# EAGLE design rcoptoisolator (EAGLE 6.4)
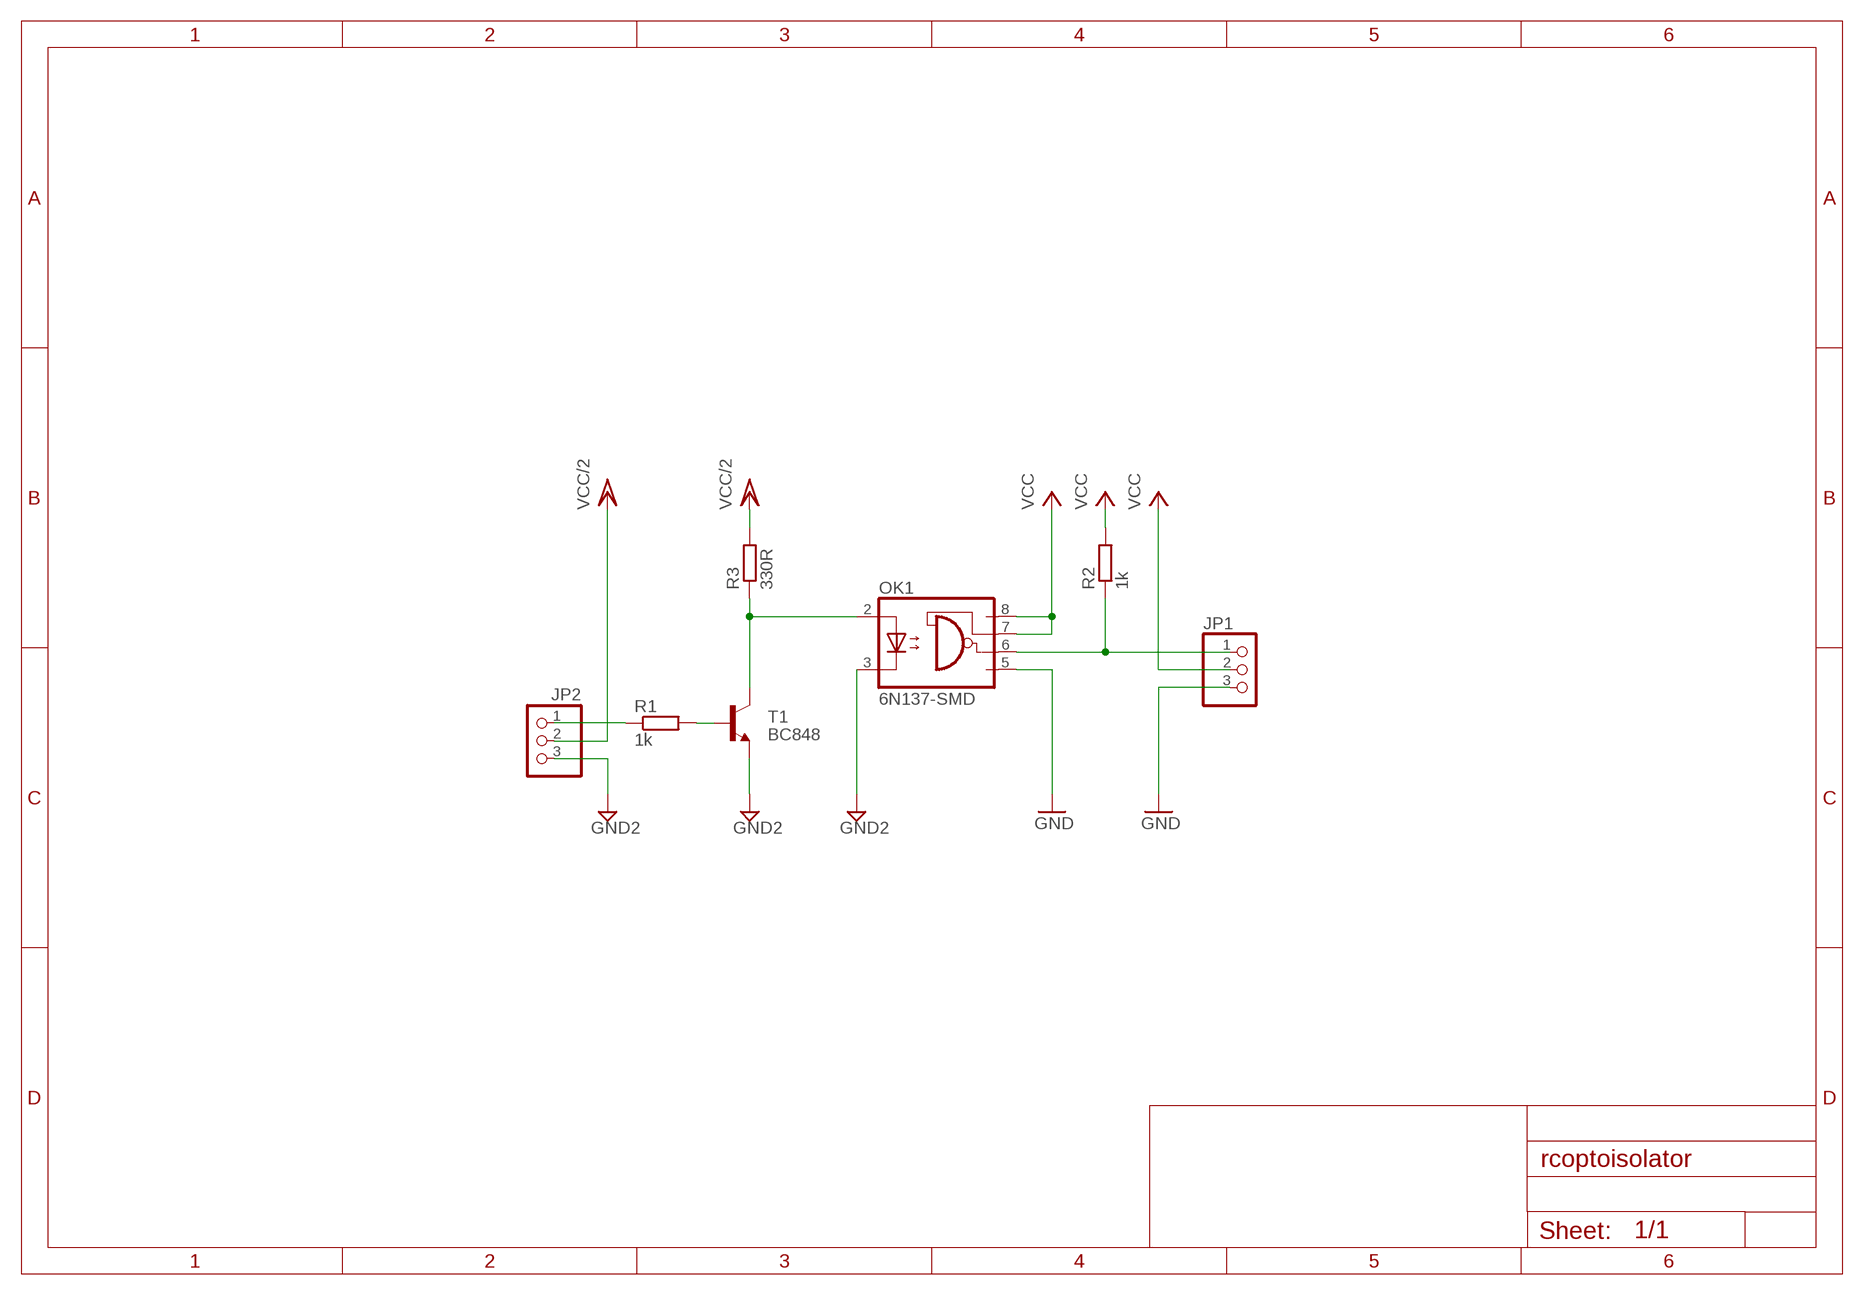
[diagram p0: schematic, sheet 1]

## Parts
JP1  PINHD-1X3  [1X03]
JP2  PINHD-1X3  [1X03]
OK1  6N137-SMD  [DIL8-SMD]
R1  1k  R-EU_KOLINM0805  [M0805]
R2  1k  R-EU_KOLINM0805  [M0805]
R3  330R  R-EU_KOLINM0805  [M0805]
T1  BC848  [SOT23]

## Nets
GND: JP1.3 OK1.5(GND)
GND2: JP2.3 OK1.3(C) T1.2(E)
N$1: JP1.1 OK1.6(VO) R2.1
N$2: R1.2 T1.1(B)
N$3: JP2.1 R1.1
N$5: OK1.2(A) R3.1 T1.3(C)
VCC: JP1.2 OK1.7(VE) OK1.8(VCC) R2.2
VCC/2: JP2.2 R3.2

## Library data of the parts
JP1 JP2 = pinhead:PINHD-1X3: PIN HEADER
OK1 = optocoupler-smd:6N137-SMD: MOTOROLA OPTO COUPLER
R1-R3 = PINHEAD_RC:R-EU_KOLIN: RESISTOR, European symbol
T1 = transistor:BC848: NPN TRANSISTOR

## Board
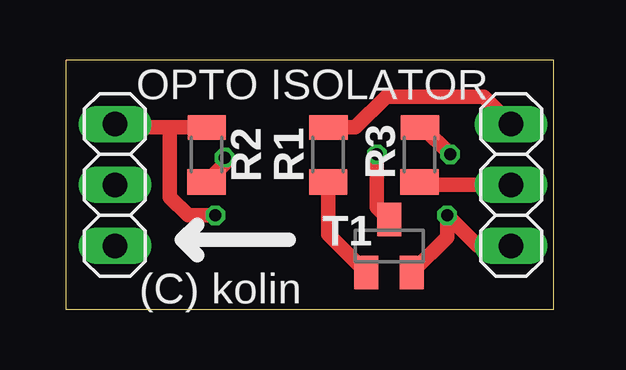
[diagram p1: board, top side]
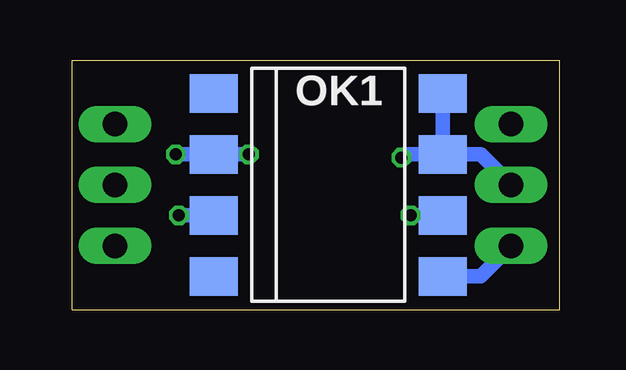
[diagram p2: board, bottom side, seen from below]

Size 20.32 x 10.41 mm. Coordinates in mm from the lower left corner, seen from the top.
Outline: 20.32,0 20.32,10.41 0,10.41 0,0 20.32,0
Copper layers (1*16): Top 0.035mm / dielectric 1.5mm / Bottom 0.035mm
Design rules "ITEADstudio_DRC": minimum track width 6mil, minimum drill 12mil, track to track 6mil, track to pad 6mil, pad to pad 6mil, via to via 6mil, smd to smd 0mil, copper to edge 10mil, drill to drill 10mil, minimum pad ring 10mil, minimum via ring 6mil, stop-mask expansion 2mil, vias tented up to drill 100mil, thermal gap 10mil

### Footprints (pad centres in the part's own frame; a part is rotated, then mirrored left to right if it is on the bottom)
1X03 = drill 1.016 long: 1 -2.54,0; 2 0,0; 3 2.54,0
DIL8-SMD = smd 1.6 x 2: 1 -3.81,-4.77; 2 -1.27,-4.77; 3 1.27,-4.77; 4 3.81,-4.77; 5 3.81,4.77; 6 1.27,4.77; 7 -1.27,4.77; 8 -3.81,4.77
M0805 = smd 1.021 x 1.6: 1 -1.131,0.017 | smd 1.046 x 1.6: 2 1.148,0
SOT23 = smd 1 x 1.4: 1 -0.95,-1.1; 2 0.95,-1.1; 3 0,1.1

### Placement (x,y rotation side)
JP1  2.03,5.21 270 top
JP2  18.54,5.21 270 top
OK1  9.65,5.21 270 bottom
R1  10.92,6.48 270 top
R2  5.84,6.48 270 top
R3  14.73,6.48 270 top
T1  13.46,2.67 0 top

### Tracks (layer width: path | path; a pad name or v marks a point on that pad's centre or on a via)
GND
  Bottom 0.61: JP1.3 3.3,1.4 OK1.5
GND2  (via drill 0.5)
  Top 0.61: JP2.3 17.14,2.67 v15.88,3.94 15.88,3.03 T1.2
  Bottom 0.61: OK1.3 v15.88,3.94
N$1  (via drill 0.5)
  Top 0.61: JP1.1 2.17,7.61 4.32,7.61 | 4.32,7.61 R2.1 | v6.22,3.94 5.08,3.94 4.32,4.7 4.32,7.61
  Bottom 0.61: OK1.6 v6.22,3.94
N$2
  Top 0.61: T1.1 10.92,3.16 R1.2
N$3
  Top 0.61: JP2.1 17.4,8.89 13.34,8.89 12.05,7.61 R1.1
N$5  (via drill 0.5)
  Top 0.61: T1.3 12.95,4.28 v12.95,6.48 | v16,6.48 14.87,7.61 R3.1
  Bottom 0.61: v12.95,6.48 OK1.2 v16,6.48
VCC  (via drill 0.5)
  Top 0.61: R2.2 6.6,6.09 v6.6,6.35
  Bottom 0.61: JP1.2 3.3,6.48 OK1.7 | v6.6,6.35 6.48,6.48 OK1.7 | OK1.8 OK1.7
VCC/2
  Top 0.61: R3.2 14.85,5.21 JP2.2

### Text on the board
tPlace: OPTO ISOLATOR | (C) kolin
